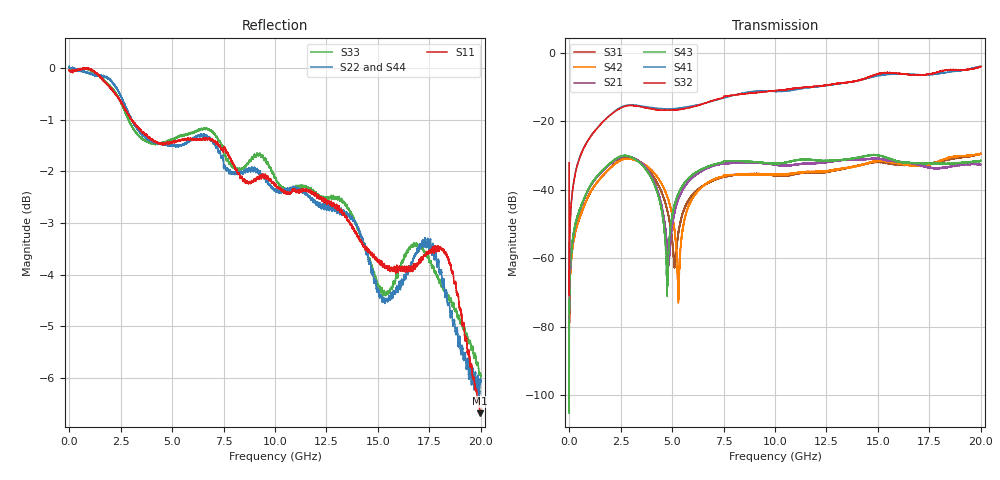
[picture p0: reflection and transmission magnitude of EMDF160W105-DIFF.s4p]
!EMDF160W105
!Johanson Technology Inc.
!www.johansontechnology.com
!Test Board Conditions:
!Substrate Type  RO4350B
!Substrate Thickness  21 mil
!Substrate Dk  3.66
!TL Type: GCPW
!TL Trace Width  40 mil
!TL Gap  17.5 mil
!PART MODE DIFFERENTIAL
!DUT TOPOLOGY	DIFFERENTIAL 4-PORT
# MHz S  dB  R 50
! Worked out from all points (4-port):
!   20001 points, 300 kHz to 20 GHz, reference 50 ohm
!   strongest paths, dB at 300 kHz, 5 GHz, 10 GHz, 15 GHz, 20 GHz:
!     S32: -32.1, -16.8, -11.1, -6.2, -4.1
!     S41: -32.1, -16.4, -11.3, -6.7, -4.0
!     S43: -84.0, -47.9, -32.3, -29.9, -31.5
!     S21: -77.5, -50.7, -32.7, -30.9, -32.7
!     S42: -86.4, -47.1, -35.6, -31.6, -29.5
!     S31: -79.7, -54.8, -35.8, -31.9, -29.4
!   lowest |S11| = -6.7 dB at 19.97 GHz (marker M1), VSWR 2.72, Z = 26.8 - j30.4 ohm
!   |S11| at or under -10 dB: nowhere
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0.3  -0.03 -178.5  -69.45 142.2  -76.57 -92.1  -32.06 -87.4
     -77.47 -6.8  0.04 -178.5  -32.18 -87.4  -84.86 -84.8
     -79.68 -88.4  -32.13 -87.3  -0.04 -178.6  -79.86 39.2
     -32.13 -87.4  -86.35 78.0  -84.01 -54.4  0.09 -178.4
2506.262  -0.64 140.3  -30.47 11.2  -31.12 1.7  -15.90 32.0
          -30.47 11.2  -0.54 142.4  -16.19 33.7  -31.41 4.6
          -31.12 1.6  -16.16 33.4  -0.65 141.6  -30.19 9.1
          -15.92 32.2  -31.40 4.4  -30.21 9.3  -0.59 141.0
4760.229  -1.45 120.4  -56.56 -73.7  -45.84 -141.4  -16.44 -12.6
          -57.39 -78.2  -1.49 116.7  -16.78 -10.3  -41.99 -126.4
          -45.77 -142.4  -16.79 -10.5  -1.41 118.6  -70.01 -38.7
          -16.41 -12.3  -41.76 -125.5  -67.94 -17.4  -1.49 115.7
5306.22  -1.40 112.4  -42.83 38.3  -52.63 40.6  -16.26 -14.7
         -42.67 37.3  -1.52 109.1  -16.56 -12.9  -72.20 124.3
         -52.93 38.0  -16.61 -12.6  -1.32 108.7  -41.25 38.7
         -16.19 -15.0  -73.07 120.5  -41.05 39.2  -1.58 106.9
7069.194  -1.41 91.8  -32.92 -10.7  -37.10 -32.9  -13.95 -23.2
          -32.90 -10.3  -1.46 95.7  -13.86 -18.0  -36.85 -33.2
          -37.11 -33.1  -13.83 -18.4  -1.28 96.1  -32.55 -11.4
          -13.97 -23.0  -36.91 -33.1  -32.59 -11.2  -1.42 91.8
19967  -6.69 -105.8  -32.88 76.7  -29.43 46.4  -4.24 143.6
       -32.62 76.3  -6.06 -104.3  -3.81 147.5  -29.60 48.8
       -29.53 46.6  -4.12 148.5  -5.91 -108.2  -31.88 71.4
       -4.03 142.7  -29.55 48.4  -31.52 70.1  -6.65 -108.9
20000  -6.67 -107.0  -32.90 75.4  -29.45 45.0  -4.15 142.8
       -32.71 74.7  -6.08 -102.6  -3.85 147.6  -29.59 48.4
       -29.41 45.2  -4.09 148.2  -5.97 -108.5  -31.82 70.0
       -3.97 142.1  -29.50 47.4  -31.50 68.5  -6.73 -109.4
